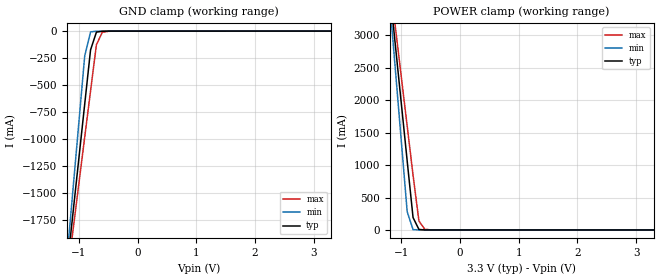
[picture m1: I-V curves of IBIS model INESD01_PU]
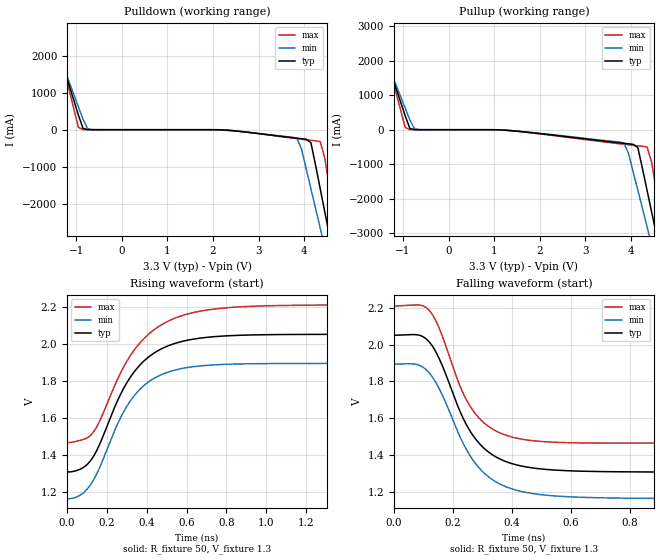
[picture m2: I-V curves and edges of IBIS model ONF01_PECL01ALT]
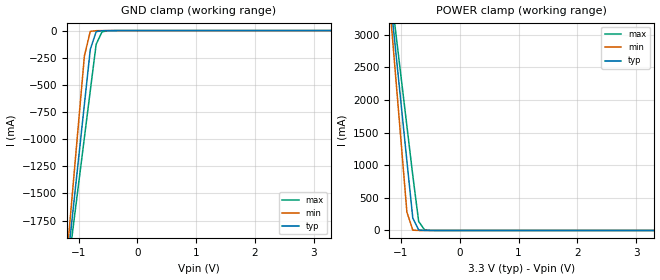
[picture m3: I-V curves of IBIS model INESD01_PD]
|   This file is an IBIS representation of the   |
|   Integrated Devices Technology, Inc.   |
|   ICS84330-01   |
|   700MHZ, LOW JITTER, CRYSTAL-TO- 3.3V LVPECL FREQUENCY SYNTHESIZER   |
[IBIS Ver]   4.1
[File name]   84330_01_3v3.ibs
[File Rev]   1.0
[Date]   13 Jan 2009 | Last modified
|   5 Dec 2002 | Generated
[Source]   Originated at Integrated Devices Technology, Inc.
[Disclaimer]
IDT hereby grants the user of this IBIS model a non-exclusive,
nontransferable license to use this IBIS model under the following terms.
Before using this IBIS model, the user should read this license.
If the user does not accept these terms,  the IBIS model should be
returned to IDT within 30 days.
   The user is granted this license only to use the IBIS model and
is not granted rights to sell, load, rent, lease or license the IBIS
model in whole or in part, or in modified form to anyone other than
user. User may modify the IBIS model to suit its specific
applications but rights to derivative works and such modifications
shall belong to IDT.
   This IBIS model is provided on an "AS IS" basis and IDT makes
absolutely no warranty with respect to the information contained
herein. IDT DISCLAIMS AND CUSTOMER WAIVES ALL WARRANTIES, EXPRESS
OR IMPLIED, INCLUDING WARRANTIES OF MERCHANTABILITY OR FITNESS FOR
A PARTICULAR PURPOSE. The entire risk as to quality and performance
is with the Customer. ACCORDINGLY, IN NO EVENT SHALL THE COMPANY BE
LIABLE FOR ANY DAMAGES, WHETHER IN CONTRACT OR TORT,INCLUDING ANY
LOST PROFITS OR OTHER INCIDENTAL, CONSEQUENTIAL, EXEMPLARY, OR
PUNITIVE DAMAGES ARISING OUT OF THE USE OR APPLICATION OF THE IBIS
model provided in this package. Further, IDT reserves the right to
make changes without notice to any product herein to improve
reliability, function, or design. IDT does not convey any license
under patent rights or any other intellectual property rights,
including those of third parties.
   IDT is not obligated to provide maintenance or support
for the licensed IBIS model.
[Copyright]   Copyright 2002 by Integrated Devices Technology, Inc.
[Component]   ICS84330M-01
[Manufacturer] Integrated Devices Technology, Inc.
[Package]
|SOIC 28 Lead
|   typ   min   max
R_pkg   57.15m   45.4m   68.9m
L_pkg   4.051nH   2.187nH   5.914nH
C_pkg   0.796pF   0.419pF   1.173pF
[Pin]   signal_name   model_name   R_pin   L_pin   C_pin
1   M0   INESD01_PU   68.9m   5.914n   1.173p
2   M1   INESD01_PU   65.0m   5.288n   1.044p
3   M2   INESD01_PU   61.1m   4.668n   0.919p
4   M3   INESD01_PU   57.2m   4.048n   0.794p
5   M4   INESD01_PU   53.2m   3.428n   0.669p
6   M5   INESD01_PU   49.3m   2.808n   0.544p
7   M6   INESD01_PU   45.4m   2.187n   0.419p
8   M7   INESD01_PU   45.4m   2.187n   0.419p
9   M8   INESD01_PU   49.3m   2.808n   0.544p
10   N0   INESD01_PU   53.2m   3.428n   0.669p
11   N1   INESD01_PU   57.2m   4.048n   0.794p
12   VEE   GND   61.1m   4.668n   0.919p
13   TEST   NC   65.0m   5.288n   1.044p
14   VCC   POWER   68.9m   5.914n   1.173p
15   VEE   GND   68.9m   5.914n   1.173p
16   nFOUT   ONF01_PECL01ALT   65.0m   5.288n   1.044p
17   FOUT   ONF01_PECL01ALT   61.1m   4.668n   0.919p
18   VCCO   POWER   57.2m   4.048n   0.794p
19   S_CLOCK   INESD01_PD   53.2m   3.428n   0.669p
20   S_DATA   INESD01_PD   49.3m   2.808n   0.544p
21   S_LOAD   INESD01_PD   45.4m   2.187n   0.419p
22   VCCA   POWER   45.4m   2.187n   0.419p
23   NC   NC   49.3m   2.808n   0.544p
24   NC   NC   53.2m   3.428n   0.669p
25   XTAL_IN   NC   57.2m   4.048n   0.794p
26   XTAL_OUT   NC   61.1m   4.668n   0.919p
27   VCC   POWER   65.0m   5.288n   1.044p
28   nP_LOAD   INESD01_PU   68.9m   5.914n   1.173p
[Diff Pin]  inv_pin  vdiff tdelay_typ tdelay_min  tdelay_max
17   16   NA   0  0  0
[Component]   ICS84330V-01
[Manufacturer] Integrated Devices Technology, Inc.
[Package]
|PLCC 28 Pin
|   typ   min   max
R_pkg   53.15m   49.2m   57.1m
L_pkg   3.123nH   2.878nH   3.368nH
C_pkg   0.65pF   0.632pF   0.667pF
[Pin]   signal_name   model_name   R_pin   L_pin   C_pin
1   VCCA   POWER   49.2m   2.878n   0.632p
2   NC   NC   51.2m   3.038n   0.643p
3   NC   NC   53.8m   3.201n   0.655p
4   XTAL_IN   NC   57.1m   3.368n   0.667p
5   XTAL_OUT   NC   57.1m   3.368n   0.667p
6   VCC   POWER   53.8m   3.201n   0.655p
7   nP_LOAD   INESD01_PU   51.2m   3.038n   0.643p
8   M0   INESD01_PU   49.2m   2.878n   0.632p
9   M1   INESD01_PU   51.2m   3.038n   0.643p
10   M2   INESD01_PU   53.8m   3.201n   0.655p
11   M3   INESD01_PU   57.1m   3.368n   0.667p
12   M4   INESD01_PU   57.1m   3.368n   0.667p
13   M5   INESD01_PU   53.8m   3.201n   0.655p
14   M6   INESD01_PU   51.2m   3.038n   0.643p
15   M7   INESD01_PU   49.2m   2.878n   0.632p
16   M8   INESD01_PU   51.2m   3.038n   0.643p
17   N0   INESD01_PU   53.8m   3.201n   0.655p
18   N1   INESD01_PU   57.1m   3.368n   0.667p
19   VEE   GND   57.1m   3.368n   0.667p
20   TEST   NC   53.8m   3.201n   0.655p
21   VCC   POWER   51.2m   3.038n   0.643p
22   VEE   GND   49.2m   2.878n   0.632p
23   nFOUT   ONF01_PECL01ALT   51.2m   3.038n   0.643p
24   FOUT   ONF01_PECL01ALT   53.8m   3.201n   0.655p
25   VCCO   POWER   57.1m   3.368n   0.667p
26   S_CLOCK   INESD01_PD   57.1m   3.368n   0.667p
27   S_DATA   INESD01_PD   53.8m   3.201n   0.655p
28   S_LOAD   INESD01_PD   51.2m   3.038n   0.643p
[Diff Pin]  inv_pin  vdiff tdelay_typ tdelay_min  tdelay_max
24   23   NA   0  0  0
| Models and submodels in the file (3): INESD01_PU (Input), ONF01_PECL01ALT (Output_ECL), INESD01_PD (Input)
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[Model]   INESD01_PU
Model_type   Input
Polarity   Non-Inverting
Vinl = 0.8V
Vinh = 2.0V
|   typ   min   max
C_comp   2pF   1.5pF   2.5pF
|   typ   min   max
[Voltage range]  3.3V   3.15V   3.45V
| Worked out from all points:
|   GND clamp passes 1 mA (typ) near -0.55 V on its own axis
|   POWER clamp passes 1 mA (typ) near -0.61 V on its own axis
[GND_clamp]
|Voltage   I(typ)   I(min)   I(max)
-3.3V     -12.83A    -15.14A    -11.37A
-1.2V     -2.195A    -2.092A    -2.281A
-1.1V     -1.689A    -1.472A    -1.849A
-900mV    -678.5mA   -232.7mA   -984.8mA
-800mV    -174mA     -7.237mA   -553.3mA
-700mV    -9.767mA   -1.114mA   -126.1mA
-600mV    -1.7mA     -240.1uA   -11.15mA
-300mV    -81.66uA   -67.79uA   -163.4uA
3.3V      1.866nA    1.113pA    239.1nA
[POWER_clamp]
|Voltage   I(typ)   I(min)   I(max)
-3.3V     22.38A     26.45A     19.82A
-1.2V     3.723A     3.545A     3.874A
-1.1V     2.836A     2.457A     3.116A
-1V       1.949A     1.369A     2.358A
-900mV    1.063A     281mA      1.601A
-800mV    191.5mA    5.012mA    843.9mA
-700mV    8.032mA    142.2uA    138.3mA
-600mV    607uA      17.63uA    10.62mA
-400mV    16.32uA    7.545uA    335.9uA
3.3V      -71.13uA   -62.11uA   -78.26uA
[Model]   ONF01_PECL01ALT
Model_type  Output_ECL
Polarity   Non-Inverting
Vmeas = 1.636
Rref = 50
Cref = 0
Vref = 1.3
|Variable  typ   min   max
C_comp   2p   1.5p   2.5p
[Voltage Range]   3.3   3.135   3.465
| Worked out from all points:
|   rising waveform, R_fixture 50, V_fixture 1.3: 20-80 % time 218ps typ, 206ps min, 242ps max; typ from 1.31 V to 2.05 V
|   falling waveform, R_fixture 50, V_fixture 1.3: 20-80 % time 134ps typ, 143ps min, 120ps max; typ from 2.05 V to 1.31 V
| Open source, no load
|  Voltage   I(typ)   I(min)   I(max)
[Pullup]
-3.3V     9.786A     8.45A      12.03A
-1.667V   3.247A     2.997A     3.691A
-1.565V   2.839A     2.657A     3.17A
-952.6mV  398mA      622.1mA    64.71mA
-850.5mV  36.63mA    284.2mA    1.532mA
-646.4mV  229.3uA    1.611mA    19.07uA
3.844V    -394.4mA   -383.6mA   -421.3mA
4.151V    -517.8mA   -1.749A    -465.4mA
4.355V    -1.764A    -2.812A    -500.3mA
4.559V    -3.036A    -3.875A    -1.773A
4.763V    -4.308A    -4.937A    -3.393A
6.6V      -15.79A    -14.52A    -18.03A
[Pulldown]
-3.3V     9.786A     8.45A      12.03A
-1.565V   2.839A     2.657A     3.17A
-1.463V   2.432A     2.317A     2.65A
-952.6mV  398mA      622.1mA    64.71mA
-850.5mV  36.63mA    284.2mA    1.532mA
-646.4mV  229.3uA    1.611mA    19.07uA
3.844V    -229.1mA   -232.1mA   -241.8mA
4.151V    -352.7mA   -1.598A    -286.7mA
4.355V    -1.599A    -2.66A     -322.1mA
4.559V    -2.871A    -3.722A    -1.595A
4.763V    -4.144A    -4.785A    -3.217A
6.6V      -15.69A    -14.41A    -17.97A
[Ramp]
|   typ   min   max
dV/dt_r   0.45V/0.37ns   0.45V/0.405ns   0.45V/0.27ns
dV/dt_f   0.45V/0.37ns   0.45V/0.405ns   0.45V/0.27ns
R_load =   50.0000
[Rising Waveform]
R_fixture = 50
V_fixture = 1.3   | VCC_typ - 2V
V_fixture_max = 1.465   | VCC_max - 2V
V_fixture_min = 1.135   | VCC_min - 2V
C_fixture = 0.0p
| Time   typ   min   max
0s        1.306V     1.161V     1.465V
70ps      1.323V     1.183V     1.479V
128ps     1.383V     1.254V     1.517V
258ps     1.703V     1.577V     1.819V
316ps     1.817V     1.689V     1.934V
398ps     1.919V     1.785V     2.042V
504ps     1.988V     1.846V     2.121V
658ps     2.03V      1.879V     2.175V
875ps     2.047V     1.891V     2.201V
2ns       2.052V     1.894V     2.211V
[Falling Waveform]
R_fixture = 50
V_fixture = 1.3   | VCC_typ - 2V
V_fixture_max = 1.465   | VCC_max - 2V
V_fixture_min = 1.135   | VCC_min - 2V
C_fixture = 0.0p
0s        2.052V     1.894V     2.211V
76ps      2.055V     1.893V     2.217V
118ps     2.018V     1.85V      2.19V
150ps     1.936V     1.772V     2.103V
222ps     1.644V     1.505V     1.782V
264ps     1.514V     1.38V      1.65V
326ps     1.409V     1.274V     1.549V
410ps     1.348V     1.21V      1.493V
708ps     1.309V     1.166V     1.465V
2ns       1.306V     1.161V     1.465V
[Model]   INESD01_PD
Model_type   Input
Polarity   Non-Inverting
Vinl = 0.80V
Vinh = 2.0V
|   typ   min   max
C_comp   2pF   1.5pF   2.5pF
|   typ   min   max
[Voltage range]  3.3V   3.15V   3.45V
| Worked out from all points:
|   GND clamp passes 1 mA (typ) near -0.55 V on its own axis
|   POWER clamp passes 1 mA (typ) near -0.60 V on its own axis
[GND_clamp]
|Voltage I(typ)   I(min)   I(max)
-3.3V     -12.83A    -15.14A    -11.37A
-1.2V     -2.195A    -2.092A    -2.281A
-1.1V     -1.689A    -1.472A    -1.849A
-900mV    -678.5mA   -232.6mA   -984.8mA
-800mV    -173.9mA   -7.175mA   -553.2mA
-700mV    -9.696mA   -1.052mA   -126mA
-600mV    -1.629mA   -178uA     -11.07mA
-300mV    -10.53uA   -5.678uA   -86.08uA
3.3V      71.13uA    62.11uA    77.58uA
[POWER_clamp]
|Voltage   I(typ)   I(min)   I(max)
-3.3V     22.38A     26.45A     19.82A
-1.2V     3.723A     3.545A     3.874A
-1.1V     2.836A     2.457A     3.116A
-1V       1.949A     1.369A     2.358A
-900mV    1.063A     281.1mA    1.601A
-800mV    191.6mA    5.074mA    844mA
-700mV    8.104mA    204.3uA    138.4mA
-600mV    678.1uA    79.74uA    10.7mA
-400mV    87.44uA    69.65uA    413.2uA
3.3V      -3.041nA   -425fA     -919.9nA
